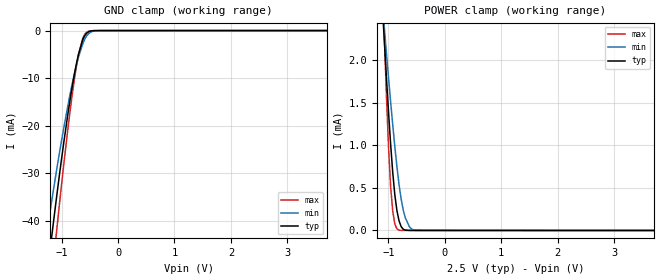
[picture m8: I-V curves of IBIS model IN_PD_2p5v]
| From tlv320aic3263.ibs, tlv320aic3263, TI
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|   IN_PD_2p5v
[Model]   IN_PD_2p5v
Model_type   Input
Vinl = 0.75
Vinh = 1.75
|   typ   min   max
C_comp   1.100pF   1.086pF   1.128pF
[Voltage Range]   2.5   2.25   2.75
[Temperature Range]   27   125   -40
[Power Clamp Reference]   2.5   2.25   2.75
[GND Clamp Reference]   -0   -0   -0
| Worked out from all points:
|   GND clamp passes 1 mA (typ) near -0.58 V on its own axis
|   POWER clamp passes 1 mA (typ) near -0.96 V on its own axis
[GND Clamp]
|   Voltage   I(typ)   I(min)   I(max)
-2.5V     -394.5mA   -329.6mA   -444mA
-1.262V   -52.04mA   -42.59mA   -62.89mA
-1.15V    -40.89mA   -33.94mA   -49.39mA
-1.113V   -37.29mA   -31.15mA   -45.01mA
-1.075V   -33.77mA   -28.41mA   -40.7mA
-887.5mV  -17.49mA   -15.72mA   -20.59mA
-737.5mV  -7.01mA    -7.302mA   -7.558mA
-700mV    -4.978mA   -5.577mA   -5.08mA
-625mV    -1.96mA    -2.786mA   -1.626mA
-550mV    -490.9uA   -1.046mA   -283uA
-325mV    -928.3nA   -10.63uA   -261.3nA
4.963V    0A         0A         0A
[POWER Clamp]
|   Voltage   I(typ)   I(min)   I(max)
-2.5V     20.66mA    14.8mA     34.71mA
-1.113V   2.682mA    2.698mA    3.063mA
-1.038V   1.815mA    2.097mA    1.618mA
-1V       1.407mA    1.805mA    1.001mA
-962.5mV  1.026mA    1.521mA    526.2uA
-925mV    689.9uA    1.247mA    232uA
-887.5mV  421.2uA    988.3uA    77.37uA
-812.5mV  114uA      540.5uA    3.857uA
-700mV    4.192uA    146.6uA    531.7nA
-625mV    522.2nA    39.4uA     513.6nA
-512.5mV  254.2nA    2.557uA    513nA
4.963V    0A         0A         0A
